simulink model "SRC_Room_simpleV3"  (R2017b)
settings: Solver=ode15s  StartTime=0.0  StopTime=tend  MaxStep=0.1  RelTol=1e-6
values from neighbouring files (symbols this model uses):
  CWlow = split(2)    [Main_Kc_v3.m]
  CWup = split(3)    [Main_Kc_v3.m]
  EHlow = split(4)    [Main_Kc_v3.m]
  EHup = split(5)    [Main_Kc_v3.m]
  HWlow = split(3)    [Main_Kc_v3.m]
  HWup = split(4)    [Main_Kc_v3.m]
  K1 = sign(Kcp(1))    [Main_Kc_v3.m]
  K2 = sign(Kcp(2))    [Main_Kc_v3.m]
  K3 = sign(Kcp(3))    [Main_Kc_v3.m]
  K4 = sign(Kcp(4))    [Main_Kc_v3.m]
  K_amb = 1    [Main_Kc_v3.m]
  K_cw = k(2)    [Main_Kc_v3.m]
  K_eh = k(4)    [Main_Kc_v3.m]
  K_hw = k(3)    [Main_Kc_v3.m]
  K_rw = k(1)    [Main_Kc_v3.m]
  Kc = double(S.Kc)    [SRC_eq_Kc_v3.m]
  Ks1 = vmax/du(1)    [Main_Kc_v3.m]
  Ks2 = vmax/du(2)    [Main_Kc_v3.m]
  Ks3 = vmax/du(3)    [Main_Kc_v3.m]
  Ks4 = vmax/du(4)    [Main_Kc_v3.m]
  Ksu = 1    [Main_Kc_v3.m]
  off1 = -split(2)    [Main_Kc_v3.m]
  off2 = 0    [Main_Kc_v3.m]
  off3 = 0    [Main_Kc_v3.m]
  off4 = -split(4)    [Main_Kc_v3.m]
  RWlow = split(1)    [Main_Kc_v3.m]
  RWup = split(2)    [Main_Kc_v3.m]
  split = split0-split0(3)*ones(1,length(split0))    [Main_Kc_v3.m]    (also in SRC_eq_Kc_v3.m)
  Tamb0 = 18    [Main_Kc_v3.m]
  Tamb1 = 2    [Main_Kc_v3.m]
  Tamb2 = 10    [Main_Kc_v3.m]
  Tamb3 = -13    [Main_Kc_v3.m]
  Tamb4 = -15    [Main_Kc_v3.m]
  tau_amb = 15    [Main_Kc_v3.m]
  tau_cw = tau(2)    [Main_Kc_v3.m]
  tau_eh = tau(4)    [Main_Kc_v3.m]
  tau_hw = tau(3)    [Main_Kc_v3.m]
  tau_rw = tau(1)    [Main_Kc_v3.m]
  tauI_sim = min(taup_tune,4*(tauc+theta))    [Main_Kc_v3.m]
  theta_amb = 6    [Main_Kc_v3.m]
  theta_cw = theta(2)    [Main_Kc_v3.m]
  theta_eh = theta(4)    [Main_Kc_v3.m]
  theta_hw = theta(3)    [Main_Kc_v3.m]
  theta_rw = theta(1)    [Main_Kc_v3.m]
  Tr0 = 18    [Main_Kc_v3.m]
  Tsp0 = 18    [Main_Kc_v3.m]
  Tsp1 = 0    [Main_Kc_v3.m]
  Tsp2 = 0    [Main_Kc_v3.m]
  Tsp3 = 0    [Main_Kc_v3.m]
  Tsp4 = 0    [Main_Kc_v3.m]
  tTamb1 = tTsp1    (= 10)    [Main_Kc_v3.m]
  tTamb2 = tTsp2    (= 60)    [Main_Kc_v3.m]
  tTamb3 = tTsp3    (= 110)    [Main_Kc_v3.m]
  tTamb4 = tTsp4    (= 160)    [Main_Kc_v3.m]
  tTsp1 = 10    [Main_Kc_v3.m]
  tTsp2 = tTsp1+50    (= 60)    [Main_Kc_v3.m]
  tTsp3 = tTsp2+50    (= 110)    [Main_Kc_v3.m]
  tTsp4 = tTsp3+50    (= 160)    [Main_Kc_v3.m]
  v10 = 0    [Main_Kc_v3.m]
  v1max = vmax    [Main_Kc_v3.m]
  v1min = 0    [Main_Kc_v3.m]
  v20 = 0    [Main_Kc_v3.m]
  v2max = vmax    [Main_Kc_v3.m]
  v2min = 0    [Main_Kc_v3.m]
  v30 = 0    [Main_Kc_v3.m]
  v3max = vmax    [Main_Kc_v3.m]
  v3min = 0    [Main_Kc_v3.m]
  v40 = 0    [Main_Kc_v3.m]
  v4max = vmax    [Main_Kc_v3.m]
  v4min = 0    [Main_Kc_v3.m]
libraries: simulink x1

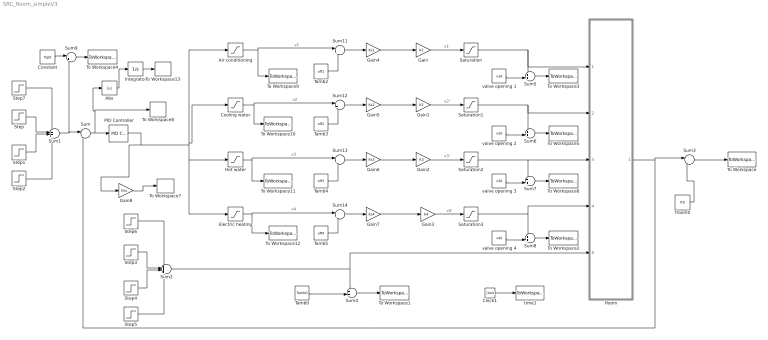
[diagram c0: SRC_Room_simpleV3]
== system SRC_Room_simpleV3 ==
  Abs : Abs
  Air conditioning : Saturate  UpperLimit=RWup  LowerLimit=RWlow
  Clock1 : Clock
  Constant : Constant  Value=Tsp0
  Cooling water : Saturate  UpperLimit=CWup  LowerLimit=CWlow
  Electric heating : Saturate  UpperLimit=EHup  LowerLimit=EHlow
  Gain : Gain  Gain=K1
  Gain1 : Gain  Gain=K2
  Gain2 : Gain  Gain=K3
  Gain3 : Gain  Gain=K4
  Gain4 : Gain  Gain=Ks1
  Gain5 : Gain  Gain=Ks2
  Gain6 : Gain  Gain=Ks3
  Gain7 : Gain  Gain=Ks4
  Gain8 : Gain  Gain=Ksu
  Hot water : Saturate  UpperLimit=HWup  LowerLimit=HWlow
  Integrator : Integrator
  PID Controller : simulink/Continuous/PID Controller  Controller=PI  TimeDomain=Continuous-time  SampleTime=-1  IntegratorMethod=Forward Euler  FilterMethod=Forward Euler  Form=Parallel  UseFilter=on  ControllerParametersSource=internal  P=Kc  I=Kc/tauI_sim  D=0  N=100  InitialConditionSource=internal  InitialConditionForIntegrator=0  InitialConditionForFilter=0  ExternalReset=none  LimitOutput=on  UpperSaturationLimit=split(5)  LowerSaturationLimit=split(1)  LinearizeAsGain=on  AntiWindupMode=back-calculation  Kb=1  TrackingMode=off  Kt=1  PParamMin=[]  PParamMax=[]  IParamMin=[]  IParamMax=[]  DParamMin=[]  DParamMax=[]  NParamMin=[]  NParamMax=[]  KbParamMin=[]  KbParamMax=[]  KtParamMin=[]  KtParamMax=[]  POutMin=[]  POutMax=[]  IOutMin=[]  IOutMax=[]  DOutMin=[]  DOutMax=[]  NOutMin=[]  NOutMax=[]  KbOutMin=[]  KbOutMax=[]  KtOutMin=[]  KtOutMax=[]  IntegratorOutMin=[]  IntegratorOutMax=[]  FilterOutMin=[]  FilterOutMax=[]  SumOutMin=[]  SumOutMax=[]  SumI1OutMin=[]  SumI1OutMax=[]  SumI2OutMin=[]  SumI2OutMax=[]  SumI3OutMin=[]  SumI3OutMax=[]  SumDOutMin=[]  SumDOutMax=[]  SaturationOutMin=[]  SaturationOutMax=[]  IntegratorContinuousStateAttributes=''  IntegratorStateMustResolveToSignalObject=off  IntegratorRTWStateStorageClass=Auto  FilterContinuousStateAttributes=''  FilterStateMustResolveToSignalObject=off  FilterRTWStateStorageClass=Auto  DifferentiatorICPrevScaledInput=0  DifferentiatorOutMin=[]  DifferentiatorOutMax=[]  InitialConditionSetting=State (most efficient)  FilterDiffOutCoefMin=[]  FilterDiffOutCoefMax=[]  SumDenOutMin=[]  SumDenOutMax=[]  SumNumOutMin=[]  SumNumOutMax=[]  ReciprocalOutMin=[]  ReciprocalOutMax=[]  DivideOutMin=[]  DivideOutMax=[]  TunerSelectOption=Transfer Function Based (PID Tuner App)
  Room : Subsystem
  Saturation : Saturate  UpperLimit=v1max  LowerLimit=v1min
  Saturation1 : Saturate  UpperLimit=v2max  LowerLimit=v2min
  Saturation2 : Saturate  UpperLimit=v3max  LowerLimit=v3min
  Saturation3 : Saturate  UpperLimit=v4max  LowerLimit=v4min
  Step : Step  Time=tTsp1  After=Tsp1  SampleTime=0
  Step1 : Step  Time=tTsp2  After=Tsp2  SampleTime=0
  Step2 : Step  Time=tTsp3  After=Tsp3  SampleTime=0
  Step3 : Step  Time=tTamb2  After=Tamb2  SampleTime=0
  Step4 : Step  Time=tTamb3  After=Tamb3  SampleTime=0
  Step5 : Step  Time=tTamb4  After=Tamb4  SampleTime=0
  Step6 : Step  Time=tTamb1  After=Tamb1  SampleTime=0
  Step7 : Step  Time=tTsp4  After=Tsp4  SampleTime=0
  Sum : Sum  Inputs=|+-
  Sum1 : Sum  Inputs=++++
  Sum{3,9,11..14} (6 alike) : Sum  Inputs=|++
  Sum2 : Sum  Inputs=++++
  Sum{4..8} (5 alike) : Sum  Inputs=++|
  Tamb0 : Constant  Value=Tamb0
  Tamb2 : Constant  Value=off1
  Tamb3 : Constant  Value=off2
  Tamb4 : Constant  Value=off3
  Tamb5 : Constant  Value=off4
  To Workspace : ToWorkspace  VariableName=Troom  SampleTime=-1
  To Workspace1 : ToWorkspace  VariableName=Tamb  SampleTime=-1
  To Workspace10 : ToWorkspace  VariableName=v2_pre  SampleTime=-1
  To Workspace11 : ToWorkspace  VariableName=v3_pre  SampleTime=-1
  To Workspace12 : ToWorkspace  VariableName=v4_pre  SampleTime=-1
  To Workspace13 : ToWorkspace  VariableName=IAE  SampleTime=-1
  To Workspace2 : ToWorkspace  VariableName=v4  SampleTime=-1
  To Workspace3 : ToWorkspace  VariableName=v1  SampleTime=-1
  To Workspace4 : ToWorkspace  VariableName=Tsp  SampleTime=-1
  To Workspace5 : ToWorkspace  VariableName=v2  SampleTime=-1
  To Workspace6 : ToWorkspace  VariableName=v3  SampleTime=-1
  To Workspace7 : ToWorkspace  VariableName=u  SampleTime=-1
  To Workspace8 : ToWorkspace  VariableName=e  SampleTime=-1
  To Workspace9 : ToWorkspace  VariableName=v1_pre  SampleTime=-1
  Troom0 : Constant  Value=Tr0
  time1 : ToWorkspace  VariableName=t  SampleTime=-1
  valve opening 1 : Constant  Value=v10
  valve opening 2 : Constant  Value=v20
  valve opening 3 : Constant  Value=v30
  valve opening 4 : Constant  Value=v40
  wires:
  Clock1/1 -> time1/1
  Sum/1 -> Abs/1, To Workspace8/1, PID Controller/1
  Step/1 -> Sum1/2
  Step1/1 -> Sum1/3
  Step2/1 -> Sum1/4
  Sum1/1 -> Sum9/2, Sum/1
  Room/1(T) -> Sum/2, Sum3/1  "T"
  Air conditioning/1 -> Sum11/1, To Workspace9/1  "v1"
  Cooling water/1 -> Sum12/1, To Workspace10/1  "v2"
  Hot water/1 -> Sum13/1, To Workspace11/1  "v3"
  Electric heating/1 -> Sum14/1, To Workspace12/1  "v4"
  Step6/1 -> Sum2/1
  Sum2/1 -> Room/5(Tamb), Sum4/1
  Step4/1 -> Sum2/3
  Step3/1 -> Sum2/2
  Step5/1 -> Sum2/4
  Troom0/1 -> Sum3/2
  Sum3/1 -> To Workspace/1
  Tamb0/1 -> Sum4/2
  Sum4/1 -> To Workspace1/1
  Saturation/1 -> Sum5/1, Room/1(vRW)
  Saturation1/1 -> Sum6/1, Room/2(vCW)
  Saturation2/1 -> Sum7/1, Room/3(vHW)
  Saturation3/1 -> Sum8/1, Room/4(vEH)
  Step7/1 -> Sum1/1
  valve opening 1/1 -> Sum5/2
  Sum5/1 -> To Workspace3/1
  Sum8/1 -> To Workspace2/1
  Sum6/1 -> To Workspace5/1
  Sum7/1 -> To Workspace6/1
  valve opening 2/1 -> Sum6/2
  valve opening 3/1 -> Sum7/2
  valve opening 4/1 -> Sum8/2
  Sum9/1 -> To Workspace4/1
  Constant/1 -> Sum9/1
  PID Controller/1 -> Gain8/1, Cooling water/1, Air conditioning/1, Electric heating/1, Hot water/1
  Gain/1 -> Saturation/1  "v1'"
  Gain1/1 -> Saturation1/1  "v2'"
  Gain2/1 -> Saturation2/1  "v3'"
  Gain3/1 -> Saturation3/1  "v4'"
  Gain4/1 -> Gain/1
  Sum11/1 -> Gain4/1
  Tamb2/1 -> Sum11/2
  Tamb3/1 -> Sum12/2
  Tamb4/1 -> Sum13/2
  Tamb5/1 -> Sum14/2
  Sum12/1 -> Gain5/1
  Gain5/1 -> Gain1/1
  Sum13/1 -> Gain6/1
  Gain6/1 -> Gain2/1
  Sum14/1 -> Gain7/1
  Gain7/1 -> Gain3/1
  Gain8/1 -> To Workspace7/1
  Integrator/1 -> To Workspace13/1
  Abs/1 -> Integrator/1

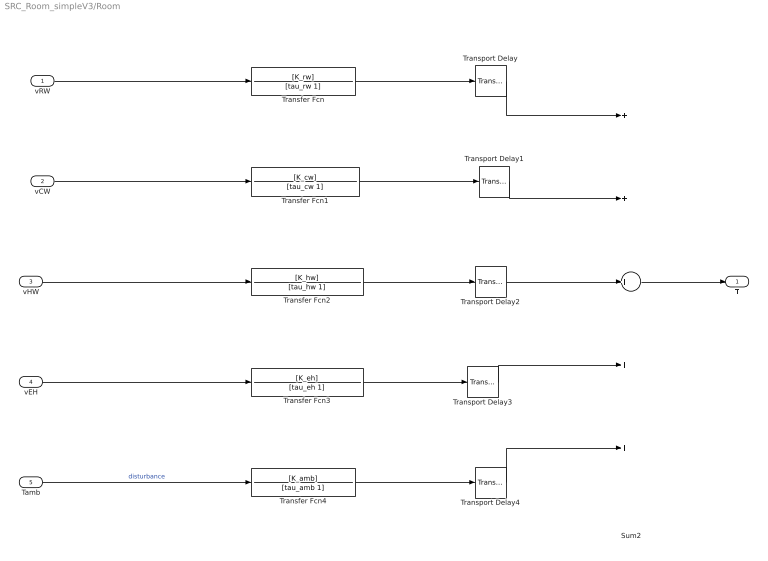
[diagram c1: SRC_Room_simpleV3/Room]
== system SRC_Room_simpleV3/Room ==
  vRW : Inport
  vCW : Inport  Port=2
  vHW : Inport  Port=3
  vEH : Inport  Port=4
  Tamb : Inport  Port=5
  Sum2 : Sum  Inputs=+++++
  Transfer Fcn : TransferFcn  Numerator=[K_rw]  Denominator=[tau_rw 1]
  Transfer Fcn1 : TransferFcn  Numerator=[K_cw]  Denominator=[tau_cw 1]
  Transfer Fcn2 : TransferFcn  Numerator=[K_hw]  Denominator=[tau_hw 1]
  Transfer Fcn3 : TransferFcn  Numerator=[K_eh]  Denominator=[tau_eh 1]
  Transfer Fcn4 : TransferFcn  Numerator=[K_amb]  Denominator=[tau_amb 1]
  Transport Delay : TransportDelay  DelayTime=theta_rw
  Transport Delay1 : TransportDelay  DelayTime=theta_cw
  Transport Delay2 : TransportDelay  DelayTime=theta_hw
  Transport Delay3 : TransportDelay  DelayTime=theta_eh
  Transport Delay4 : TransportDelay  DelayTime=theta_amb
  T : Outport
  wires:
  vRW/1 -> Transfer Fcn/1
  vCW/1 -> Transfer Fcn1/1
  vHW/1 -> Transfer Fcn2/1
  vEH/1 -> Transfer Fcn3/1
  Sum2/1 -> T/1
  Tamb/1 -> Transfer Fcn4/1  "disturbance"
  Transfer Fcn/1 -> Transport Delay/1
  Transfer Fcn1/1 -> Transport Delay1/1
  Transfer Fcn2/1 -> Transport Delay2/1
  Transfer Fcn3/1 -> Transport Delay3/1
  Transfer Fcn4/1 -> Transport Delay4/1
  Transport Delay/1 -> Sum2/1
  Transport Delay1/1 -> Sum2/2
  Transport Delay2/1 -> Sum2/3
  Transport Delay3/1 -> Sum2/4
  Transport Delay4/1 -> Sum2/5
